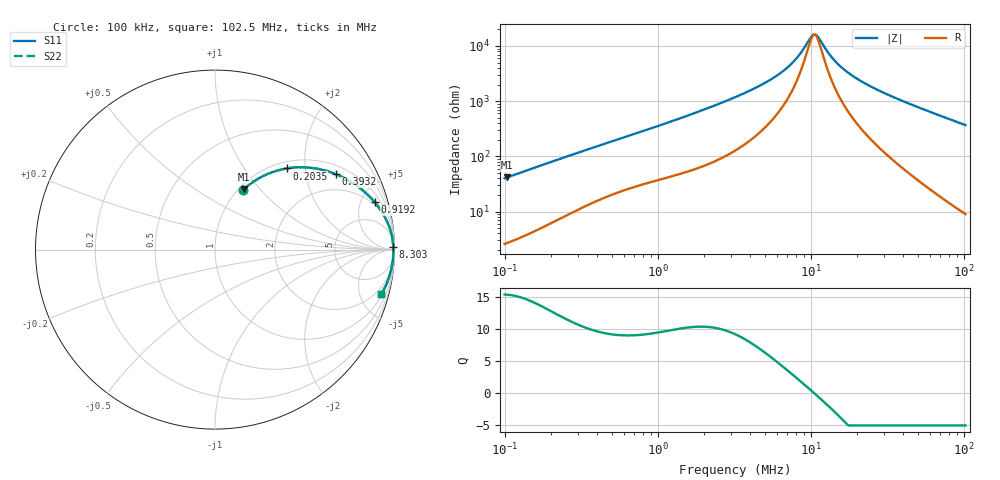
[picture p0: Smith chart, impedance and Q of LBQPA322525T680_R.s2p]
! LBQPA322525T680_R  S-PARAMETER MODEL  ( General Type )
! Model Generated by TAIYO YUDEN Corporation (http://www.ty-top.com)
! Version 1.0
! TAIYO YUDEN Control No. 191025NI43SB-FBB
! Copyright(c) 2019 TAIYO YUDEN CO.,LTD. All Rights Reserved.
! Product Description (link to TY-COMPAS)
! https://ds.yuden.co.jp/TYCOMPAS/or/detail?pn=LBQPA322525T680KR&u=M
! Products Name : Inductors
! Characteristics :
!  Inductance : 68 uH , SRF(min) : 8.0 MHz , DC Resistance(max) : 1.3 Ohm
!  Rated Current : Saturation :320 mA , Temp Rise : 260 mA (20 degC)
!  Case Size : 3.2 x 2.5 / 0.126 x 0.098 [mm/inch] , Thickness : 2.5 / 0.098 [mm/inch]
!  (Conditions: Temperature = 25 degC , DC Bias Current/Voltage = 0A / 0V)
! External Node Assignments :
!  1  o---GGG---o  2
! GND o---------o GND
! Frequency Range : 0.1MHz  -  102.47202MHz  [ 402 STEP ]
# MHz S RI R 50
! Freq[MHz].  S11 Real  S11 Imag  S21 Real  S21 Imag  S12 Real  S12 Imag  S22 Real  S22 Imag
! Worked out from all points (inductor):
!   401 points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, 100 kHz to 102.5 MHz, reference 50 ohm
!   read as one part in series: L = 63.3 uH near 103.5 kHz
!   highest Q = 15.4 at 103.5 kHz (marker M1), where L = 63.5 uH
!   self-resonance near 10.58 MHz
!   S11 on the Smith chart (normalised r, x): 100 kHz: 1.05, +0.80; 203.5 kHz: 1.13, +1.60; 393.2 kHz: 1.30, +2.96; 919.2 kHz: 1.69, +6.48; 8.303 MHz: open; 102.5 MHz: 1.18, -7.37
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0.1  0.1535 0.3295  0.8465 -0.3295  0.8465 -0.3295  0.1535 0.3295
0.103527  0.1618 0.3373  0.8382 -0.3373  0.8382 -0.3373  0.1618 0.3373
0.203511  0.3986 0.452  0.6014 -0.452  0.6014 -0.452  0.3986 0.452
0.319357  0.5928 0.446  0.4072 -0.446  0.4072 -0.446  0.5928 0.446
0.393183  0.6732 0.4206  0.3268 -0.4206  0.3268 -0.4206  0.6732 0.4206
0.595979  0.8014 0.3476  0.1986 -0.3476  0.1986 -0.3476  0.8014 0.3476
0.919165  0.8906 0.2632  0.1094 -0.2632  0.1094 -0.2632  0.8906 0.2632
1.019889  0.9063 0.2437  0.0937 -0.2437  0.0937 -0.2437  0.9063 0.2437
1.9033  0.9649 0.1423  0.0351 -0.1423  0.0351 -0.1423  0.9649 0.1423
3.257086  0.9844 0.0807  0.0156 -0.0807  0.0156 -0.0807  0.9844 0.0807
4.527234  0.9897 0.053  0.0103 -0.053  0.0103 -0.053  0.9897 0.053
5.871251  0.992 0.0348  0.00804 -0.0348  0.00804 -0.0348  0.992 0.0348
7.104316  0.993 0.0229  0.00704 -0.0229  0.00704 -0.0229  0.993 0.0229
8.303494  0.9935 0.0137  0.00653 -0.0137  0.00653 -0.0137  0.9935 0.0137
10.22302  0.9938 0.00195  0.00617 -0.00195  0.00617 -0.00195  0.9938 0.00195
10.58357  0.9939 1.15e-05  0.00615 -1.15e-05  0.00615 -1.15e-05  0.9939 1.15e-05
11.14838  0.9939 -0.0029  0.00613 0.0029  0.00613 0.0029  0.9939 -0.0029
13.72555  0.9938 -0.0147  0.00625 0.0147  0.00625 0.0147  0.9938 -0.0147
17.1939  0.9932 -0.0282  0.00677 0.0282  0.00677 0.0282  0.9932 -0.0282
22.68813  0.9919 -0.0468  0.00815 0.0468  0.00815 0.0468  0.9919 -0.0468
32.64791  0.9881 -0.0768  0.0119 0.0768  0.0119 0.0768  0.9881 -0.0768
102.472  0.9261 -0.2496  0.0739 0.2496  0.0739 0.2496  0.9261 -0.2496
